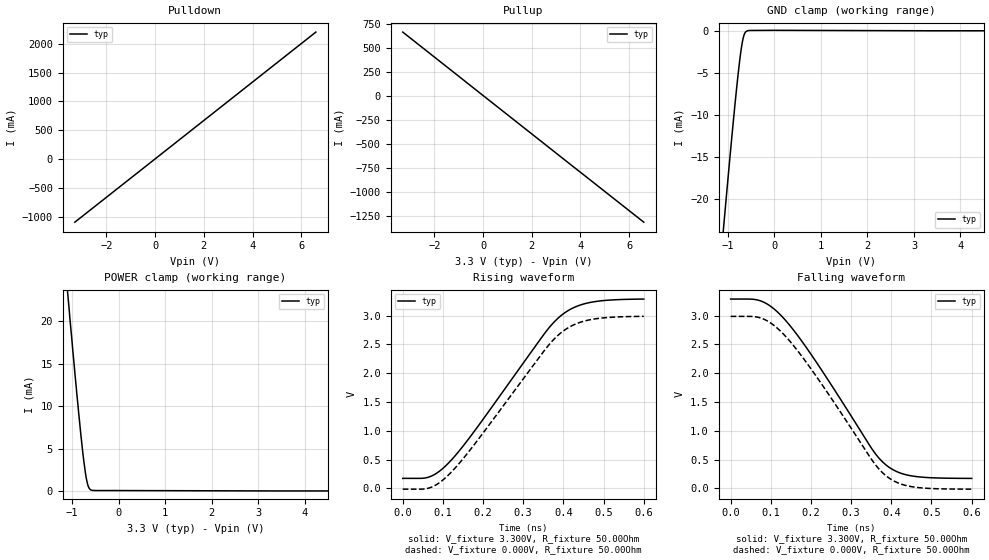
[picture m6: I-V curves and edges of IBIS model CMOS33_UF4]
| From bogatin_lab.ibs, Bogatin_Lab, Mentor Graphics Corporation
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[Model]   CMOS33_UF4
Model_type   I/O
Vinl = 800.000mV
Vinh = 2.000V
Vmeas = 1.500V
Vref = 0.000V
Cref = 50.000pF
Rref = 1.000kOhm
|   typ   min   max
C_comp   4.000pF   NA   NA
[Voltage Range]   3.300V   NA   NA
[Temperature Range]   50.0   NA   NA
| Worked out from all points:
|   slope of the pulldown table from 0 to 0.495 V, typ, clamps not added: 3 ohm
|   slope of the pullup table from 0 to 0.495 V, typ, clamps not added: 5 ohm
|   GND clamp passes 1 mA (typ) near -0.68 V on its own axis
|   POWER clamp passes 1 mA (typ) near -0.68 V on its own axis
|   falling waveform, V_fixture 3.300V, R_fixture 50.00Ohm: 20-80 % time 176ps typ, NA min, NA max; typ from 3.29 V to 0.175 V
|   rising waveform, V_fixture 3.300V, R_fixture 50.00Ohm: 20-80 % time 193ps typ, NA min, NA max; typ from 0.175 V to 3.29 V
|   rising waveform, V_fixture 0.000V, R_fixture 50.00Ohm: 20-80 % time 193ps typ, NA min, NA max; typ from -0.012 V to 2.99 V
|   falling waveform, V_fixture 0.000V, R_fixture 50.00Ohm: 20-80 % time 176ps typ, NA min, NA max; typ from 2.99 V to -0.012 V
[Pulldown]
|   Voltage   I(typ)   I(min)   I(max)
-3.3V     -1.095A    NA         NA
5.11V     1.709A     NA         NA
5.13V     1.712A     NA         NA
6.6V      2.205A     NA         NA
[GND Clamp]
|   Voltage   I(typ)   I(min)   I(max)
-3.3V     -166.6mA   NA         NA
-1.09V    -23.21mA   NA         NA
-1.08V    -22.59mA   NA         NA
-970mV    -15.86mA   NA         NA
-850mV    -8.86mA    NA         NA
-800mV    -6.155mA   NA         NA
-750mV    -3.695mA   NA         NA
-710mV    -2.035mA   NA         NA
-670mV    -834.6uA   NA         NA
-630mV    -223.2uA   NA         NA
-590mV    -22.7uA    NA         NA
6.6V      0A         NA         NA
[Pullup]
|   Voltage   I(typ)   I(min)   I(max)
-3.3V     663.5mA    NA         NA
-1.83V    368.2mA    NA         NA
-1.81V    366.2mA    NA         NA
6.6V      -1.316A    NA         NA
[POWER Clamp]
|   Voltage   I(typ)   I(min)   I(max)
-3.3V     166.5mA    NA         NA
-1.09V    23.07mA    NA         NA
-1.08V    22.46mA    NA         NA
-940mV    13.9mA     NA         NA
-860mV    9.29mA     NA         NA
-810mV    6.549mA    NA         NA
-750mV    3.621mA    NA         NA
-710mV    2.008mA    NA         NA
-670mV    867.1uA    NA         NA
-630mV    294.2uA    NA         NA
-590mV    105.4uA    NA         NA
6.6V      0A         NA         NA
[Ramp]
R_load = 50.00Ohm
|   typ   min   max
dV/dt_r   1.799V/193.410ps   NA   NA
dV/dt_f   1.867V/175.821ps   NA   NA
[Falling Waveform]
V_fixture = 3.300V
R_fixture = 50.00Ohm
|   Time   V(typ)   V(min)   V(max)
0s        3.287V     NA         NA
74.3ps    3.255V     NA         NA
100.7ps   3.155V     NA         NA
129ps     2.976V     NA         NA
205.3ps   2.275V     NA         NA
354.9ps   656.2mV    NA         NA
391ps     385.4mV    NA         NA
420.4ps   273.2mV    NA         NA
456.5ps   211.6mV    NA         NA
600.2ps   174.6mV    NA         NA
[Rising Waveform]
V_fixture = 3.300V
R_fixture = 50.00Ohm
|   Time   V(typ)   V(min)   V(max)
0s        174.6mV    NA         NA
65.5ps    199.2mV    NA         NA
88.96ps   287mV      NA         NA
114.4ps   444.4mV    NA         NA
176.9ps   980.4mV    NA         NA
356.8ps   2.723V     NA         NA
399.8ps   3.03V      NA         NA
432.1ps   3.157V     NA         NA
470.2ps   3.232V     NA         NA
600.2ps   3.287V     NA         NA
[Rising Waveform]
V_fixture = 0.000V
R_fixture = 50.00Ohm
|   Time   V(typ)   V(min)   V(max)
0s        -12.24mV   NA         NA
66.48ps   10.12mV    NA         NA
89.94ps   93.6mV     NA         NA
115.4ps   244.3mV    NA         NA
178.9ps   768.6mV    NA         NA
358.8ps   2.448V     NA         NA
400.8ps   2.737V     NA         NA
433.1ps   2.861V     NA         NA
471.2ps   2.934V     NA         NA
600.2ps   2.987V     NA         NA
[Falling Waveform]
V_fixture = 0.000V
R_fixture = 50.00Ohm
|   Time   V(typ)   V(min)   V(max)
0s        2.987V     NA         NA
75.27ps   2.957V     NA         NA
101.7ps   2.861V     NA         NA
130ps     2.689V     NA         NA
206.3ps   2.015V     NA         NA
355.8ps   455.2mV    NA         NA
393ps     187.9mV    NA         NA
422.3ps   81.27mV    NA         NA
458.5ps   22.89mV    NA         NA
600.2ps   -12.24mV   NA         NA
